FUNCTION_BLOCK FB_Writer
VAR_INPUT
	bWrite		: BOOL;		(* Rising edge starts program execution*)
	sNetId		: T_AmsNetId := '';	(* TwinCAT system network address *)
	sFileName	: T_MaxString;		(*  := 'HardDisk\TextModeGen.csv' CSV destination file path and name*) 
	pBuffer		: POINTER TO T_Buffer;
END_VAR
VAR_OUTPUT
	bBusy: BOOL; 
	bError			: BOOL;
	nErrId			: UDINT;
END_VAR
VAR  
	fbFileOpen	: FB_FileOpen;(* Opens file *)
	fbFileClose	: FB_FileClose;(* Closes file *)
	fbAdsRdWrt	: FW_AdsRdWrt := ( nPort := AMSPORT_R3_SYSSERV, nIdxGrp := SYSTEMSERVICE_FPUTS, cbReadLen := 0, pReadBuff := 0 );	(* Writes one record (line) *)

 	_hFile			: UINT		:= 0;(* File handle of the source file *)
	_iStep			: DWORD 	:= 0;

	_iLen1: UDINT;
	_iLen2: UDINT;
	
	_iRow: UDINT;
	_iLastRow: UDINT;
	
	_iCol: UDINT;
	_iLastCol: UDINT;
	
	_iOffset: UDINT;
	
	_iCpy: UDINT;
	_pBuffer: PVOID;
	_sBuffer: STRING(MAX_BEFFER_SIZE);
END_VAR
 
VAR CONSTANT
	cs_Seperator: STRING[1]:= ';'; (*CSV字段分隔符*)
	cs_CarriageReturn: STRING[2]:= '$R$N'; (*回车换行符*)
	
	MAX_BEFFER_SIZE:UINT := 8192;(*每条ADS写命令写下去的内存大小*)
END_VAR

CASE _iStep OF
	0:	(* Wait for rising edge at bWrite variable *)
		IF bWrite THEN
			bWrite 		:= FALSE;
			bBusy 		:= TRUE;
			bError		:= FALSE;
			nErrId		:= 0;
			_hFile		:= 0; 
			_iStep 		:= 1;
			_iLastRow 	:= 0;
			_iLastCol   := 0;
		END_IF

	1:	(* Open source file *)
		fbFileOpen(  bExecute := FALSE  );
		fbFileOpen( 	sNetId := sNetId, sPathName := sFileName, nMode := FOPEN_MODEWRITE OR FOPEN_MODETEXT,(* Open file in TEXT mode! *)
						ePath := PATH_GENERIC, bExecute := TRUE );
		_iStep := 2;

	2:(* Wait until open not busy *)
		fbFileOpen( bExecute := FALSE, bError => bError, nErrID => nErrID, hFile => _hFile );
		IF NOT fbFileOpen.bBusy THEN
			IF NOT fbFileOpen.bError THEN
				_iStep := 3;
			ELSE(* Error: file not found? *)
				_iStep := 100;
			END_IF
		END_IF

	3:(* Convert one PLC record to CSV format *) 
		MEMSET(ADR(_sBuffer),0,MAX_BEFFER_SIZE);
		_iOffset := 0;
		_iCpy := 0;
		_pBuffer := ADR(_sBuffer);
		FOR _iRow := _iLastRow TO MAX_CSV_ROWS BY 1 DO
			FOR _iCol := _iLastCol TO MAX_CSV_COLUMNS BY 1 DO 
				_iLen1 := LEN(pBuffer^[ _iRow, _iCol]);
				_iLen2 := LEN(cs_Seperator); 
				IF (_iOffset + _iLen1 + _iLen2 + 1) < MAX_BEFFER_SIZE THEN 
					_iCpy := FW_MemCpy(_pBuffer + _iOffset, ADR(pBuffer^[ _iRow, _iCol]), _iLen1);
					_iOffset := _iOffset + _iCpy;
					IF  _iCol < MAX_CSV_COLUMNS THEN
						_iCpy := FW_MemCpy(_pBuffer + _iOffset, ADR(cs_Seperator), _iLen2);
						_iOffset := _iOffset + _iCpy;
					END_IF
				ELSE
					_iLastRow := _iRow;
					_iLastCol := _iCol;
					_iStep := 4;(* Write record to the file *)
					RETURN;	
				END_IF
			END_FOR 
			_iLen2 := LEN(cs_CarriageReturn); 
			_iCpy:= FW_MemCpy(_pBuffer + _iOffset, ADR(cs_CarriageReturn), _iLen2);
			_iOffset := _iOffset + _iCpy;
			_iLastCol := 0;
		END_FOR 
		_iStep := 4;(* Write record to the file *) 
	4:	(* Write single text line *) 
		fbAdsRdWrt( bExecute := FALSE ); 
		fbAdsRdWrt( sNetId := sNetId, nIdxOffs := _hFile, cbWriteLen := _iOffset + 1(*inclusive terminating NULL*), pWriteBuff := ADR(_sBuffer),
			bExecute := TRUE, tTimeout := DEFAULT_ADS_TIMEOUT, bBusy=>bBusy, bError=>bError, nErrID=>nErrID );
		_iStep := 5;

	5:(* Wait until write not busy *)
		fbAdsRdWrt( bExecute := FALSE, bError => bError, nErrID => nErrID );
		IF NOT fbAdsRdWrt.bBusy THEN
			IF NOT fbAdsRdWrt.bError THEN 
				_iStep := 3;(* Write next record *)
				IF _iRow >= MAX_CSV_ROWS THEN
					_iStep := 10;
				END_IF
			ELSE(* Error *)
				_iStep := 100;
			END_IF
		END_IF

	10:	(* Close source file *)
		fbFileClose( bExecute := FALSE );
		fbFileClose( sNetId := sNetId, hFile := _hFile, bExecute := TRUE );
		_iStep := 11;

	11:(* Wait until close not busy *)
		fbFileClose( bExecute := FALSE, bError => bError, nErrID => nErrID );
		IF ( NOT fbFileClose.bBusy ) THEN
			_hFile := 0;
			_iStep := 100;
		END_IF

	100: (* Error or ready step => cleanup *)
		IF ( _hFile <> 0 ) THEN
			_iStep := 10; (* Close the source file *)
		ELSE
			bBusy := FALSE;
			_iStep := 0;	(* Ready *) 
		END_IF

END_CASE

END_FUNCTION_BLOCK
